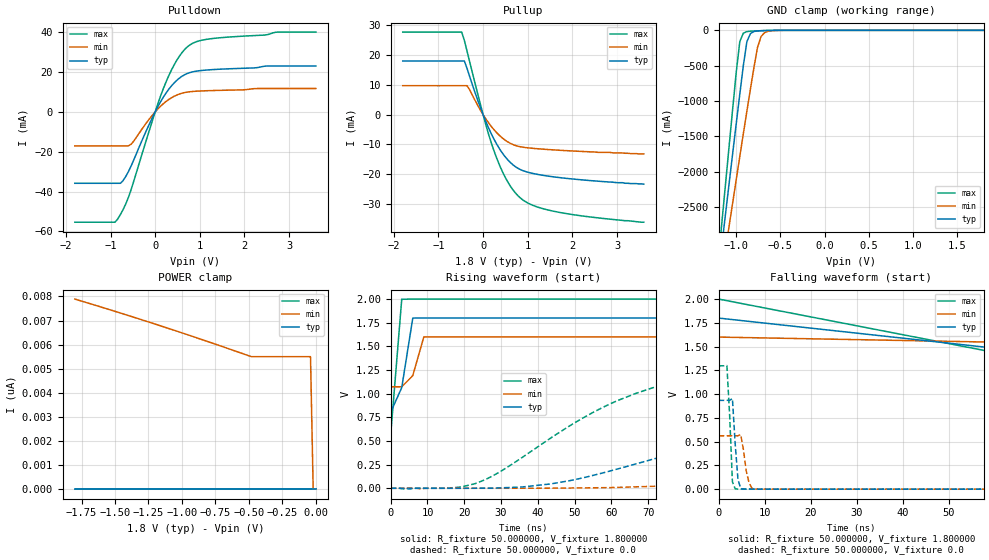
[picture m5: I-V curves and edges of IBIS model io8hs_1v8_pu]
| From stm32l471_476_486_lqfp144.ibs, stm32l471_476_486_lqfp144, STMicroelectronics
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|   Model io8hs_1v8_pu
[Model]  io8hs_1v8_pu
Model_type I/O
Polarity   Non-Inverting
Enable   Active-Low
Vinl =   0.540000V
Vinh =   1.260000V
Vmeas =  0.900000V
Cref =   100.000000nF
Rref =   1.000000k
Vref =   1.800000V
C_comp   2.197300pF   2.162700pF   2.264100pF
[Temperature Range]   25.000000   0.125000k   -40.000000
[Pullup Reference]   1.800000V   1.600000V   2.000000V
[Pulldown Reference]   0.0V   0.0V   0.0V
[POWER Clamp Reference]   1.800000V   1.600000V   2.000000V
[GND Clamp Reference]   0.0V   0.0V   0.0V
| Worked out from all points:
|   slope of the pulldown table from 0 to 0.27 V, typ, clamps not added: 26.2 ohm
|   slope of the pullup table from 0 to 0.27 V, typ, clamps not added: 30.1 ohm
|   GND clamp passes 1 mA (typ) near -0.58 V on its own axis
|   rising waveform, R_fixture 50.000000, V_fixture 1.800000: 20-80 % time 2.89ns typ, 2.56ns min, 1.8ns max; typ from 0.804 V to 1.8 V
|   rising waveform, R_fixture 50.000000, V_fixture 0.0: 20-80 % time 64.8ns typ, 104ns min, 36.2ns max; typ from 0 V to 0.934 V
|   falling waveform, R_fixture 50.000000, V_fixture 1.800000: 20-80 % time 116ns typ, 164ns min, 92ns max; typ from 1.8 V to 0.804 V
|   falling waveform, R_fixture 50.000000, V_fixture 0.0: 20-80 % time 808ps typ, 1.12ns min, 746ps max; typ from 0.934 V to 0 V
[Pulldown]
|Voltage   I(typ)   I(min)   I(max)
-1.8V     -35.82mA   -17.03mA   -55.34mA
-900mV    -35.82mA   -17.03mA   -55.34mA
-840mV    -35.82mA   -17.03mA   -53.76mA
-720mV    -34.49mA   -17.03mA   -49.08mA
-540mV    -27.18mA   -16.22mA   -39.07mA
-60mV     -2.756mA   -1.584mA   -4.227mA
240mV     9.353mA    5.171mA    14.85mA
480mV     15.75mA    8.427mA    25.77mA
720mV     19.29mA    9.947mA    32.62mA
960mV     20.57mA    10.43mA    35.5mA
1.32V     21.27mA    10.74mA    36.91mA
3.6V      23.03mA    11.73mA    40.05mA
[Pullup]
|Voltage   I(typ)   I(min)   I(max)
-1.8V     18.05mA    9.741mA    27.78mA
-480mV    18.05mA    9.741mA    27.78mA
-420mV    18.05mA    9.741mA    25.03mA
-360mV    15.57mA    9.741mA    21.38mA
60mV      -2.268mA   -1.401mA   -3.341mA
240mV     -8.143mA   -5.004mA   -12mA
360mV     -11.31mA   -6.914mA   -16.72mA
540mV     -15mA      -9.056mA   -22.31mA
840mV     -18.52mA   -10.83mA   -28.11mA
1.14V     -19.87mA   -11.38mA   -30.67mA
1.68V     -21.13mA   -11.96mA   -32.81mA
3.6V      -23.4mA    -13.2mA    -36.2mA
[GND_clamp]
|Voltage   I(typ)   I(min)   I(max)
-1.8V     -9.861A    -8.8A      -9.626A
-1.16V    -3.004A    -3.417A    -2.68A
-1.12V    -2.579A    -3.088A    -2.15A
-1.08V    -2.155A    -2.76A     -1.623A
-1V       -1.315A    -2.108A    -586.3mA
-960mV    -900.6mA   -1.784A    -158.3mA
-920mV    -496.8mA   -1.462A    -39.39mA
-880mV    -160.5mA   -1.144A    -17.82mA
-840mV    -45.92mA   -830.3mA   -12.52mA
-760mV    -8.262mA   -243mA     -7.547mA
-680mV    -3.389mA   -33.05mA   -3.833mA
1.8V      0A         0A         0A
[POWER_clamp]
|Voltage   I(typ)   I(min)   I(max)
-1.8V     0A         7.891nA    0A
-1.14V    0A         6.744nA    0A
-480mV    0A         5.5nA      0A
-40mV     0A         5.5nA      0A
-20mV     0A         0A         0A
0V        0A         0A         0A
[Ramp]
| variable   typ   min   max
dV/dt_r  0.56066/65.10411n   0.33689/0.11591u   0.77868/36.15625n
dV/dt_f  0.59736/66.12115n   0.31662/0.11582u   0.86072/35.01231n
R_load = 50.000000
[Rising Waveform]
R_fixture= 50.000000
V_fixture= 1.800000
V_fixture_min= 1.600000
V_fixture_max= 2.000000
|time   V(typ)   V(min)   V(max)
0s        804.4mV    1.072V     565.5mV
3.003ns   1.063V     1.072V     1.998V
6.006ns   1.799V     1.191V     2V
9.009ns   1.8V       1.599V     2V
297.3ns   1.8V       1.6V       2V
[Rising Waveform]
R_fixture= 50.000000
V_fixture= 0.0
V_fixture_min= 0.0
V_fixture_max= 0.0
|time   V(typ)   V(min)   V(max)
0s        2.064nV    42.97nV    1.55nV
23.42ns   438.5uV    -34.28uV   54.81mV
43.24ns   44.83mV    999.1uV    524.4mV
61.26ns   199.9mV    9.048mV    920mV
76.88ns   366.4mV    29.79mV    1.123V
91.89ns   517mV      65.46mV    1.214V
121.9ns   732.6mV    173.7mV    1.276V
156.8ns   854.3mV    302.9mV    1.292V
224ns     923.9mV    479.8mV    1.298V
299.1ns   934.4mV    561.5mV    1.298V
[Falling Waveform]
R_fixture= 50.000000
V_fixture= 1.800000
V_fixture_min= 1.600000
V_fixture_max= 2.000000
|time   V(typ)   V(min)   V(max)
0s        1.8V       1.6V       2V
150.2ns   1.008V     1.466V     594.5mV
300.3ns   817.6mV    1.137V     566.2mV
450.5ns   805.6mV    1.084V     565.5mV
750.8ns   804.4mV    1.073V     565.5mV
14.86us   804.4mV    1.072V     565.5mV
[Falling Waveform]
R_fixture= 50.000000
V_fixture= 0.0
V_fixture_min= 0.0
V_fixture_max= 0.0
|time   V(typ)   V(min)   V(max)
0s        934.4mV    561.5mV    1.298V
1.802ns   934.6mV    561.5mV    1.3V
2.402ns   934.5mV    561.5mV    772.3mV
3.003ns   952.8mV    561.7mV    78.1mV
3.604ns   478.8mV    561.7mV    4.018mV
4.204ns   104.1mV    561.4mV    1.327mV
4.805ns   5.772mV    574.5mV    885.1uV
6.607ns   524.2uV    69.78mV    483.8uV
7.808ns   310.3uV    1.813mV    360uV
299.1ns   2.064nV    42.97nV    1.55nV
